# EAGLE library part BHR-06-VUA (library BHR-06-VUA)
Box Header, Vertical, 6 Pos Source: Datasheet
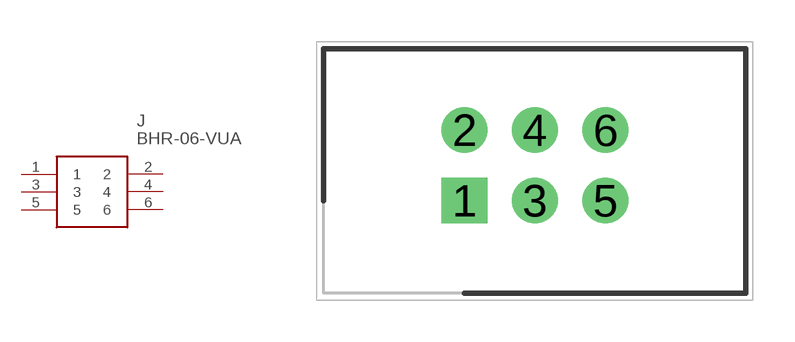
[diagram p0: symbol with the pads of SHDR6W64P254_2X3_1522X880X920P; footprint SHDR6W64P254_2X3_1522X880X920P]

Designator prefix J

## BHR-06-VUA (Description: Box Header, Vertical, 6 Pos; Height: 9.2mm; Manufacturer_Name: Adam Tech; Manufacturer_Part_Number: BHR-06-VUA)  [SHDR6W64P254_2X3_1522X880X920P]
1  1
2  2
3  3
4  4
5  5
6  6

## Footprint SHDR6W64P254_2X3_1522X880X920P (pad centres in mm)
BHR-06-VUA
drill 1.1 pad 1.65 square: 1 0,0
drill 1.1 pad 1.65: 2 0,2.54; 3 2.54,0; 4 2.54,2.54; 5 5.08,0; 6 5.08,2.54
